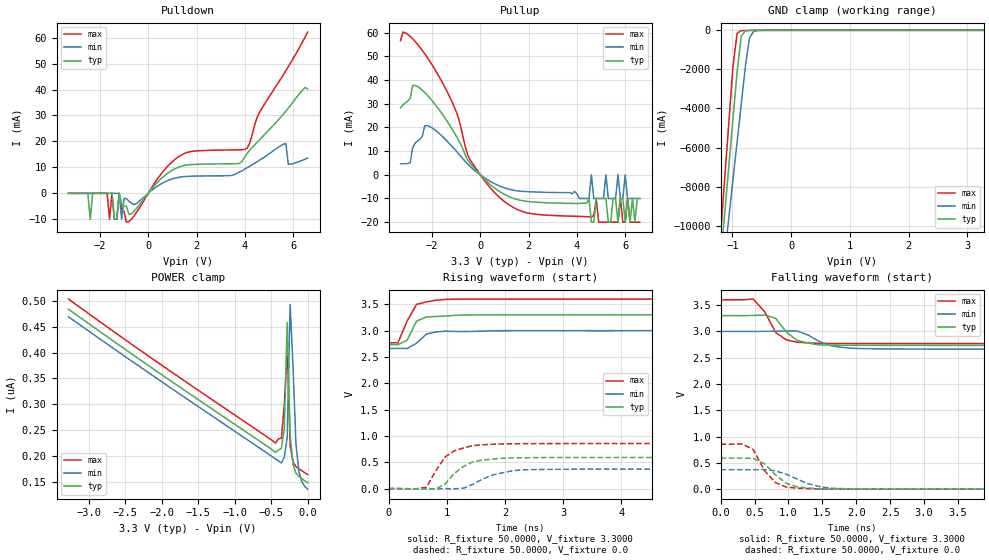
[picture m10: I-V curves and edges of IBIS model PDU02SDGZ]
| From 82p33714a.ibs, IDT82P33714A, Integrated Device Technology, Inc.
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|   Model PDU02SDGZ
[Model]  PDU02SDGZ
Model_type I/O
Polarity   Non-Inverting
Enable   Active-Low
Vinl =   0.8000V
Vinh =   2.0000V
Vmeas =  1.6500V
Cref =   50.0000pF
Rref =   1.0000M
Vref =   0.0V
C_comp   2.6301pF   2.6149pF   2.6344pF
[Temperature Range]   25.0000   0.1250k   -40.0000
[Voltage Range]   3.3000V   3.0000V   3.6000V
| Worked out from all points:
|   slope of the pulldown table from 0 to 0.495 V, typ, clamps not added: 93.5 ohm
|   slope of the pullup table from 0 to 0.495 V, typ, clamps not added: 103 ohm
|   GND clamp passes 1 mA (typ) near -0.64 V on its own axis
|   rising waveform, R_fixture 50.0000, V_fixture 3.3000: 20-80 % time 160ps typ, 217ps min, 223ps max; typ from 2.73 V to 3.3 V
|   rising waveform, R_fixture 50.0000, V_fixture 0.0: 20-80 % time 387ps typ, 506ps min, 360ps max; typ from 0.002 V to 0.591 V
|   falling waveform, R_fixture 50.0000, V_fixture 3.3000: 20-80 % time 262ps typ, 328ps min, 254ps max; typ from 3.3 V to 2.73 V
|   falling waveform, R_fixture 50.0000, V_fixture 0.0: 20-80 % time 304ps typ, 439ps min, 267ps max; typ from 0.591 V to 0.002 V
[Pulldown]
|Voltage   I(typ)   I(min)   I(max)
-3.3V     0A         0A         0A
-2.5V     0A         0A         0A
-2.4V     -10mA      0A         0A
-1.6V     0A         0A         -10mA
-1.5V     0A         0A         0A
-1.4V     -10mA      0A         -10mA
-1.2V     0A         0A         0A
-1.1V     -4mA       -10mA      -6mA
-900mV    -5mA       -2mA       -11.12mA
1.3V      10.23mA    6.236mA    14.34mA
4.1V      15.46mA    9.888mA    17.41mA
6.6V      40.22mA    13.56mA    62.13mA
[Pullup]
|Voltage   I(typ)   I(min)   I(max)
-3.3V     28.25mA    4.655mA    56.59mA
-2.2V     33.66mA    20.75mA    49.56mA
-400mV    4.59mA     3.281mA    5.938mA
1V        -8.271mA   -5.504mA   -11.3mA
4.5V      -10mA      -10mA      -17.71mA
4.6V      -20mA      0A         -18mA
4.7V      -20mA      -10mA      -17mA
4.8V      -10mA      -10mA      -10mA
6V        -20mA      0A         -20mA
6.1V      -10mA      -10mA      -10mA
6.2V      -20mA      -10mA      -20mA
6.6V      -10mA      -10mA      -20mA
[GND_clamp]
|Voltage   I(typ)   I(min)   I(max)
-3.3V     -83.46A    -71.04A    -95.7A
-1.2V     -11.69A    -13.39A    -10.37A
-1.13V    -9.3A      -11.47A    -7.522A
-1.06V    -6.904A    -9.549A    -4.675A
-990mV    -4.509A    -7.624A    -1.828A
-920mV    -2.113A    -5.699A    -140.8mA
-850mV    -308.3mA   -3.775A    -17.67mA
-780mV    -30.2mA    -1.85A     -8.762mA
-710mV    -4.268mA   -388.3mA   -4.618mA
-640mV    -880.5uA   -62.96mA   -1.8mA
-430mV    -65.09uA   -278uA     -100.1uA
3.28V     145.9nA    236.1nA    133.9nA
[POWER_clamp]
|Voltage   I(typ)   I(min)   I(max)
-3.28V    484.3nA    469.6nA    504nA
-440mV    206.6nA    193.8nA    224.5nA
-400mV    211.3nA    189.9nA    232.8nA
-360mV    214.2nA    185.9nA    233.8nA
-320mV    252.2nA    197.2nA    299.4nA
-280mV    458.6nA    236.1nA    406nA
-240mV    241nA      493.7nA    220.6nA
-200mV    183.2nA    373.1nA    187.4nA
-160mV    166.5nA    222.6nA    179.2nA
-120mV    159.8nA    169.6nA    174.8nA
-80mV     155.4nA    149.7nA    171nA
0V        147.8nA    135.2nA    163.6nA
[Ramp]
| variable   typ   min   max
dV/dt_r  0.3537/0.3867n   0.2215/0.4958n   0.5121/0.3601n
dV/dt_f  0.3396/0.2623n   0.2022/0.3186n   0.4986/0.2510n
R_load = 50.0000
[Rising Waveform]
R_fixture= 50.0000
V_fixture= 3.3000
V_fixture_min= 3.0000
V_fixture_max= 3.6000
L_fixture= 0.0H
C_fixture= 0.0F
|time   V(typ)   V(min)   V(max)
0s        2.734V     2.663V     2.769V
160ps     2.734V     2.663V     2.768V
320ps     2.82V      2.662V     3.188V
480ps     3.181V     2.762V     3.499V
650ps     3.261V     2.936V     3.546V
810ps     3.269V     2.975V     3.578V
970ps     3.276V     2.99V      3.593V
1.29ns    3.296V     2.983V     3.599V
1.62ns    3.3V       2.992V     3.599V
16ns      3.3V       3V         3.6V
[Rising Waveform]
R_fixture= 50.0000
V_fixture= 0.0
V_fixture_min= 0.0
V_fixture_max= 0.0
L_fixture= 0.0H
C_fixture= 0.0F
|time   V(typ)   V(min)   V(max)
0s        1.872mV    1.272mV    2.628mV
650ps     -91.22uV   -3.843mV   27.13mV
810ps     -5.889mV   -843uV     338.4mV
970ps     87.9mV     235.8uV    601.6mV
1.13ns    290.1mV    -3.465mV   718.1mV
1.29ns    423mV      9.865mV    774.9mV
1.62ns    544.1mV    183.7mV    833.5mV
2.1ns     583.8mV    333.7mV    851.8mV
2.59ns    589.3mV    363.5mV    855.1mV
16ns      591.4mV    370.5mV    856.2mV
[Falling Waveform]
R_fixture= 50.0000
V_fixture= 3.3000
V_fixture_min= 3.0000
V_fixture_max= 3.6000
L_fixture= 0.0H
C_fixture= 0.0F
|time   V(typ)   V(min)   V(max)
0s        3.3V       3V         3.6V
480ps     3.302V     2.999V     3.614V
650ps     3.311V     3V         3.372V
810ps     3.248V     3.004V     2.98V
970ps     2.985V     3.007V     2.837V
1.13ns    2.827V     3.007V     2.794V
1.45ns    2.744V     2.809V     2.773V
1.78ns    2.737V     2.698V     2.77V
2.59ns    2.734V     2.665V     2.769V
16ns      2.734V     2.663V     2.769V
[Falling Waveform]
R_fixture= 50.0000
V_fixture= 0.0
V_fixture_min= 0.0
V_fixture_max= 0.0
L_fixture= 0.0H
C_fixture= 0.0F
|time   V(typ)   V(min)   V(max)
0s        591.4mV    370.5mV    856.2mV
320ps     591.7mV    370.4mV    859.3mV
480ps     585.8mV    370.5mV    751.4mV
650ps     481.8mV    373.1mV    348.5mV
810ps     268.8mV    348mV      124.2mV
970ps     110.6mV    284.7mV    39.2mV
1.29ns    21.59mV    102.1mV    11.59mV
1.62ns    5.536mV    20.14mV    3.057mV
2.26ns    1.803mV    1.8mV      2.717mV
16ns      1.864mV    1.264mV    2.626mV
